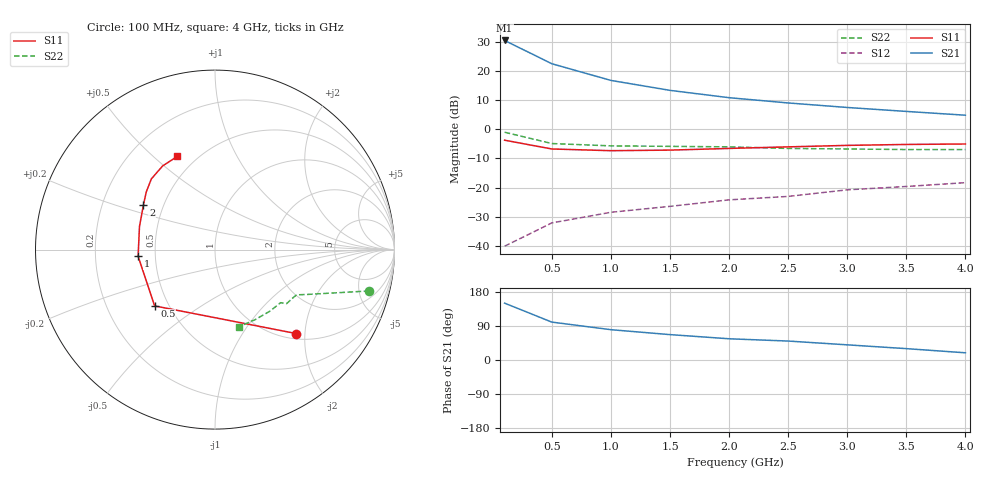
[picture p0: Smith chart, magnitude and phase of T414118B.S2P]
!AT-41411
!S-PARAMETERS at Vce=8V  Ic=25mA.  LAST UPDATED 07-21-92
# ghz s ma r 50
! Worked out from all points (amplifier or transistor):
!   9 points, 100 MHz to 4 GHz, reference 50 ohm
!   highest |S21| = 30.4 dB at 100 MHz (marker M1)
!   |S21| within 3 dB of that: start of sweep to 250.6 MHz
!   unconditionally stable (mu >= 1): 905.7 MHz to end of sweep
!   at 500 MHz: K = 0.77, MSG = 27.2 dB, |S12| = -32.0 dB
!   at 2 GHz: K = 1.23, MAG = 14.6 dB, |S12| = -24.2 dB
!   at 4 GHz: K = 1.18, MAG = 8.9 dB, |S12| = -18.3 dB
!   S11 on the Smith chart (normalised r, x): 100 MHz: 1.11, -1.80; 500 MHz: 0.42, -0.33; 1 GHz: 0.40, -0.04; 2 GHz: 0.39, +0.25; 4 GHz: 0.40, +0.60
0.1  0.65 -46.0  33.07 150.0  0.01 59.0  0.89 -15.0
0.5  0.46 -137.0  13.21 100.0  0.025 56.0  0.57 -26.0
1  0.43 -175.0  6.85 80.0  0.038 58.0  0.52 -29.0
1.5  0.44 163.0  4.63 67.0  0.048 61.0  0.51 -32.0
2  0.47 148.0  3.47 56.0  0.062 61.0  0.5 -37.0
2.5  0.5 140.0  2.82 50.0  0.071 60.0  0.47 -39.0
3  0.53 132.0  2.36 40.0  0.092 61.0  0.46 -48.0
3.5  0.55 122.0  2.02 30.0  0.105 57.0  0.45 -60.0
4  0.56 112.0  1.74 19.0  0.122 53.0  0.45 -73.0
